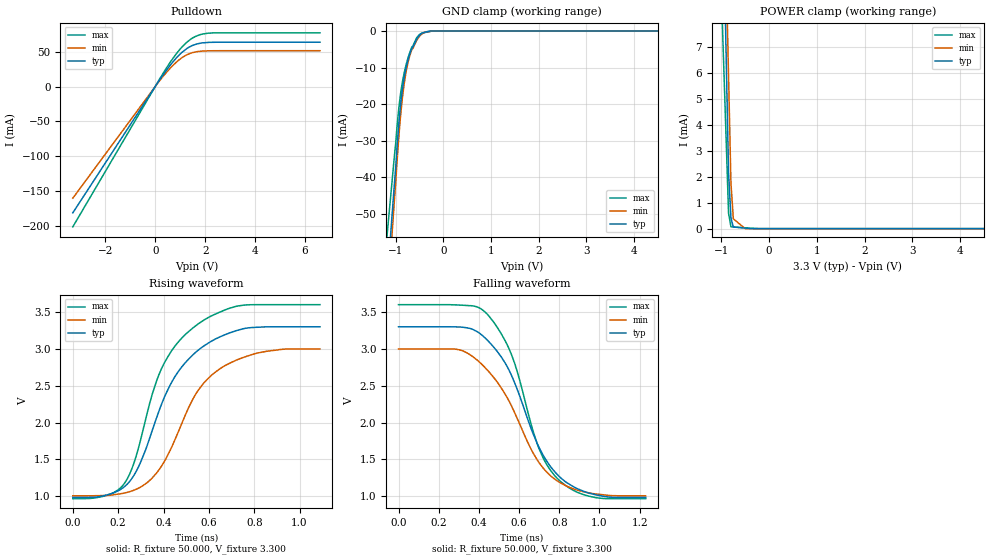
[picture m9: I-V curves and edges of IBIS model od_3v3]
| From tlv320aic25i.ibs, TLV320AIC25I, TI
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[Model]   od_3v3
Model_type I/O_open_drain
Vinl=9.900E-01
Vinh=2.310E+00
Vref=3.300E+00
Rref=5.000E+02
Cref=2.000E-11
Vmeas=1.650E+00
C_comp   1.070E-12   1.070E-12   1.070E-12
[Voltage Range]   3.300E+00   3.000E+00   3.600E+00
[POWER Clamp Reference]   3.300E+00   3.000E+00   3.600E+00
[GND Clamp Reference]   0.000E+00   0.000E+00   0.000E+00
[Pullup Reference]   3.300E+00   3.000E+00   3.600E+00
[Pulldown Reference]   0.000E+00   0.000E+00   0.000E+00
[Temperature Range]   25   85   -40
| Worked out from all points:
|   slope of the pulldown table from 0 to 0.495 V, typ, clamps not added: 19.3 ohm
|   GND clamp passes 1 mA (typ) near -0.49 V on its own axis
|   POWER clamp passes 1 mA (typ) near -0.82 V on its own axis
|   rising waveform, R_fixture 50.000, V_fixture 3.300: 20-80 % time 207ps typ, 207ps min, 186ps max; typ from 0.985 V to 3.3 V
|   falling waveform, R_fixture 50.000, V_fixture 3.300: 20-80 % time 221ps typ, 237ps min, 187ps max; typ from 3.3 V to 0.985 V
[GND Clamp]
-3.3V     -442.3mA   -468.4mA   -354mA
-1.02V    -40.48mA   -44.95mA   -33.16mA
-940mV    -26.26mA   -30.01mA   -21.75mA
-900mV    -20.47mA   -23.54mA   -17.31mA
-860mV    -16mA      -18.37mA   -13.92mA
-780mV    -9.824mA   -11mA      -9.125mA
-720mV    -6.907mA   -7.44mA    -6.427mA
-660mV    -4.67mA    -4.99mA    -4.318mA
-560mV    -2.165mA   -2.517mA   -1.838mA
-460mV    -610.5uA   -873.5uA   -677.3uA
-240mV    0A         0A         0A
6.6V      0A         0A         0A
[POWER Clamp]
-3.3V     220.2mA    206.7mA    138.1mA
-1.1V     24.4mA     26.34mA    14.62mA
-850mV    2.148mA    5.848mA    588.7uA
-800mV    406.3uA    1.75mA     70.76uA
-750mV    62.13uA    376.4uA    64.33uA
-500mV    20.71uA    0A         32.16uA
-200mV    0A         0A         0A
6.6V      0A         0A         0A
[Pulldown]
-3.3V     -181.7mA   -160.6mA   -201.9mA
200mV     10.99mA    9.561mA    12.37mA
620mV     31.68mA    27.24mA    36.04mA
860mV     41.73mA    35.54mA    47.88mA
1.08V     49.52mA    41.81mA    57.28mA
1.34V     56.37mA    46.84mA    65.93mA
1.52V     59.54mA    49.11mA    70.41mA
1.78V     62.24mA    50.68mA    74.51mA
2.16V     63.63mA    51.46mA    76.93mA
6.6V      63.85mA    51.62mA    77.36mA
[Rising Waveform]
R_fixture = 50.000
V_fixture = 3.300
V_fixture_min = 3.000
V_fixture_max = 3.600
|  time   V(typ)   V(min)   V(max)
0s        984.8mV    1.008V     968.5mV
150ps     1.019V     1.012V     1.014V
230ps     1.137V     1.047V     1.186V
300ps     1.47V      1.128V     1.779V
390ps     2.24V      1.405V     2.724V
450ps     2.622V     1.765V     3.036V
530ps     2.921V     2.322V     3.285V
610ps     3.102V     2.638V     3.446V
730ps     3.255V     2.859V     3.583V
1.09ns    3.3V       3V         3.6V
[Falling Waveform]
R_fixture = 50.000
V_fixture = 3.300
V_fixture_min = 3.000
V_fixture_max = 3.600
|  time   V(typ)   V(min)   V(max)
0s        3.3V       3V         3.6V
300ps     3.297V     2.989V     3.595V
420ps     3.176V     2.776V     3.525V
490ps     2.97V      2.555V     3.298V
550ps     2.712V     2.293V     3.002V
590ps     2.457V     2.061V     2.7V
690ps     1.719V     1.496V     1.714V
780ps     1.326V     1.229V     1.273V
950ps     1.042V     1.046V     1.001V
1.23ns    984.8mV    1.008V     968.5mV
[Ramp]
dV/dt_r   1.389E+00/2.063E-10   1.195E+00/2.071E-10   1.579E+00/1.855E-10
dV/dt_f   1.389E+00/2.206E-10   1.195E+00/2.362E-10   1.579E+00/1.871E-10
R_load = 50
